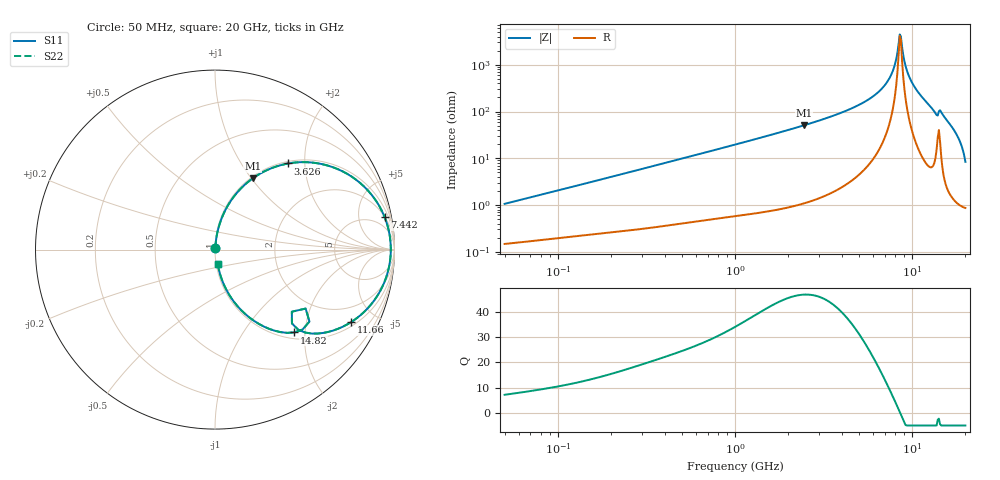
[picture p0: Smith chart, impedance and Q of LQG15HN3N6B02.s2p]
!Murata Part Number: LQG15HN3N6B02
!These Parameters are Measured in Series Mode Connection
!  o--[Z]--o
!Port1  Port2
!  o-------o
!Freq. Start=50[MHz] Stop=20[GHz], 401[Steps]
# Hz S RI R 50
!Freq.(Hz) S11(Real) S11(Imag) S21(Real) S21(Imag) S12(Real) S12(Imag) S22(Real) S22(Imag)
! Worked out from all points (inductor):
!   401 points, 50 MHz to 20 GHz, reference 50 ohm
!   read as one part in series: L = 3.31 nH near 51.52 MHz
!   highest Q = 46.8 at 2.456 GHz (marker M1), where L = 3.29 nH
!   self-resonance near 8.516 GHz
!   S11 on the Smith chart (normalised r, x): 50 MHz: 1.00, +0.02; 3.626 GHz: 1.04, +1.65; 7.442 GHz: 2, +10; 11.66 GHz: 1.18, -3.65; 14.82 GHz: 1.13, -1.76; 20 GHz: 1.02, -0.17
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5e7  0.00158 0.0105  0.9984 -0.0105  0.9984 -0.0105  0.00158 0.0105
1.364002e8  0.00298 0.0274  0.997 -0.0274  0.997 -0.0274  0.00298 0.0274
3.721004e8  0.00874 0.0726  0.9913 -0.0726  0.9913 -0.0726  0.00874 0.0726
1e9  0.0421 0.1866  0.9579 -0.1866  0.9579 -0.1866  0.0421 0.1866
2.456456e9  0.2105 0.3971  0.7895 -0.3971  0.7895 -0.3971  0.2105 0.3971
2.728004e9  0.253 0.4241  0.747 -0.4241  0.747 -0.4241  0.253 0.4241
3.626126e9  0.4077 0.4798  0.5923 -0.4798  0.5923 -0.4798  0.4077 0.4798
5.769027e9  0.7716 0.3998  0.2284 -0.3998  0.2284 -0.3998  0.7716 0.3998
6.701223e9  0.8856 0.2883  0.1144 -0.2883  0.1144 -0.2883  0.8856 0.2883
7.442007e9  0.9456 0.1796  0.0544 -0.1796  0.0544 -0.1796  0.9456 0.1796
7.901521e9  0.9679 0.1071  0.0321 -0.1071  0.0321 -0.1071  0.9679 0.1071
8.389408e9  0.9788 0.0284  0.0212 -0.0284  0.0212 -0.0284  0.9788 0.0284
8.644534e9  0.9793 -0.0127  0.0207 0.0127  0.0207 0.0127  0.9793 -0.0127
9.178299e9  0.9694 -0.0972  0.0306 0.0972  0.0306 0.0972  0.9694 -0.0972
9.600142e9  0.9515 -0.1611  0.0485 0.1611  0.0485 0.1611  0.9515 -0.1611
1.034674e10  0.9 -0.2644  0.1 0.2644  0.1 0.2644  0.9 -0.2644
1.166392e10  0.7588 -0.4036  0.2412 0.4036  0.2412 0.4036  0.7588 -0.4036
1.354865e10  0.4643 -0.4468  0.5357 0.4468  0.5357 0.4468  0.4643 -0.4468
1.417136e10  0.5049 -0.3286  0.4951 0.3286  0.4951 0.3286  0.5049 -0.3286
1.482269e10  0.4426 -0.4614  0.5574 0.4614  0.5574 0.4614  0.4426 -0.4614
1.774144e10  0.1089 -0.2949  0.8911 0.2949  0.8911 0.2949  0.1089 -0.2949
2e10  0.0153 -0.0814  0.9847 0.0814  0.9847 0.0814  0.0153 -0.0814
